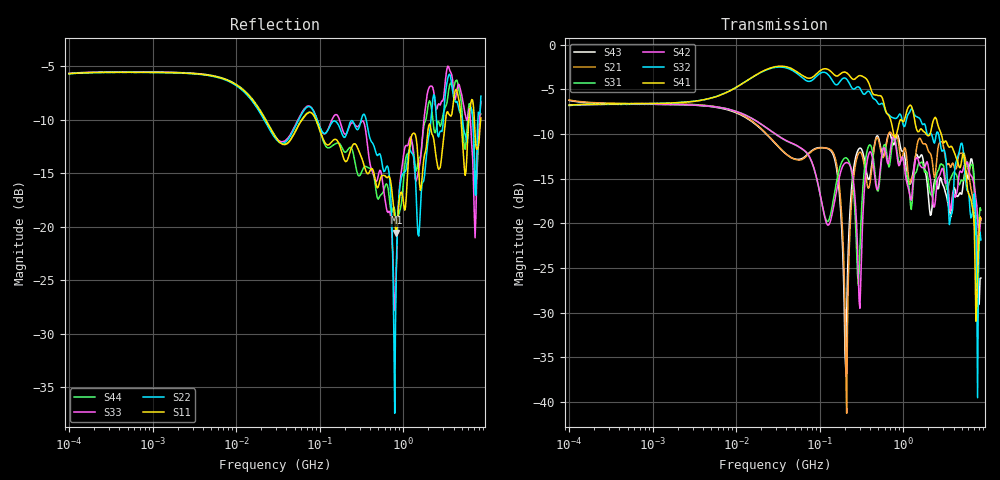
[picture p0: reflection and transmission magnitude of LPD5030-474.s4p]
# MHz S MA R 50
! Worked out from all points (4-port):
!   498 points, 100 kHz to 8.5 GHz, reference 50 ohm
!   strongest paths, dB at 100 kHz, 1.698 MHz, 29.49 MHz, 500.7 MHz, 8.5 GHz:
!     S41: -6.8, -6.5, -2.5, -5.7, -19.5
!     S32: -6.8, -6.6, -2.6, -6.6, -21.9
!     S42: -6.8, -6.7, -10.0, -16.0, -19.4
!     S31: -6.8, -6.7, -10.0, -16.4, -18.5
!     S21: -6.2, -6.6, -11.0, -10.5, -19.7
!     S43: -6.3, -6.7, -11.1, -10.3, -26.1
!   lowest |S11| = -20.6 dB at 827.5 MHz (marker M1), VSWR 1.21, Z = 46.1 - j8.16 ohm
!   |S11| at or under -10 dB: 90.34 MHz to 3.214 GHz (3.123 GHz wide, 189 % of centre); 4.917 GHz to 6.098 GHz (1.181 GHz wide, 21.4 % of centre); 7.103 GHz to 8.465 GHz (1.362 GHz wide, 17.5 % of centre)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
0.1  0.5187 8.7  0.4893 -9.9  0.4561 -170.2  0.4585 10.4
     0.4893 -9.9  0.5169 8.6  0.4574 10.4  0.4563 -170.4
     0.4561 -170.2  0.4574 10.4  0.521 8.7  0.4868 -10.0
     0.4585 10.4  0.4563 -170.4  0.4868 -10.0  0.5198 8.8
136.2065  0.2466 -32.0  0.2574 30.5  0.1141 168.5  0.7064 -27.7
          0.2574 30.5  0.3009 -21.2  0.6472 -32.1  0.1051 168.2
          0.1141 168.5  0.6472 -32.1  0.3076 -19.9  0.2541 29.3
          0.7064 -27.7  0.1051 168.2  0.2541 29.3  0.236 -31.9
210.2067  0.2021 -39.3  0.008649 54.6  0.2315 31.3  0.6943 -41.5
          0.008649 54.6  0.2722 -29.4  0.6398 -44.1  0.2186 33.1
          0.2315 31.3  0.6398 -44.1  0.2731 -35.7  0.03044 81.5
          0.6943 -41.5  0.2186 33.1  0.03044 81.5  0.2248 -41.4
276.4819  0.2388 -54.0  0.2286 39.0  0.07023 -24.1  0.6536 -51.0
          0.2286 39.0  0.2854 -45.7  0.5764 -52.9  0.09789 -36.0
          0.07023 -24.1  0.5764 -52.9  0.2938 -50.5  0.2447 33.3
          0.6536 -51.0  0.09789 -36.0  0.2447 33.3  0.1832 -57.4
827.4608  0.09362 -110.6  0.3134 -97.9  0.2692 -107.4  0.312 -122.3
          0.3134 -97.9  0.06556 -45.5  0.3867 -126.5  0.2572 -109.1
          0.2692 -107.4  0.3867 -126.5  0.0648 -48.8  0.3058 -101.0
          0.312 -122.3  0.2572 -109.1  0.3058 -101.0  0.1041 -96.9
4484.409  0.4155 -167.2  0.2213 153.1  0.1767 131.5  0.2196 112.1
          0.2213 153.1  0.375 180.0  0.2353 134.9  0.158 154.4
          0.1767 131.5  0.2353 134.9  0.4511 -179.7  0.1413 155.1
          0.2196 112.1  0.158 154.4  0.1413 155.1  0.4697 179.5
8500  0.3217 -10.1  0.104 -0.3  0.1186 -25.4  0.1062 2.5
      0.104 -0.3  0.4073 -23.2  0.08075 -26.2  0.1066 -23.6
      0.1186 -25.4  0.08075 -26.2  0.3849 -27.7  0.04939 -4.6
      0.1062 2.5  0.1066 -23.6  0.04939 -4.6  0.336 -31.8
